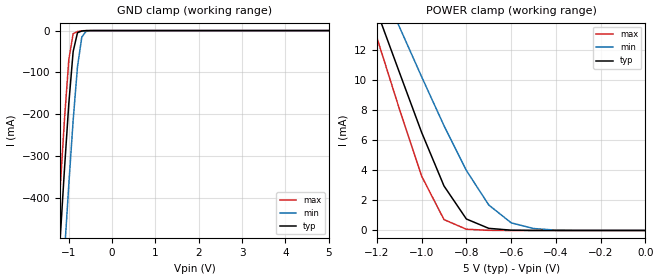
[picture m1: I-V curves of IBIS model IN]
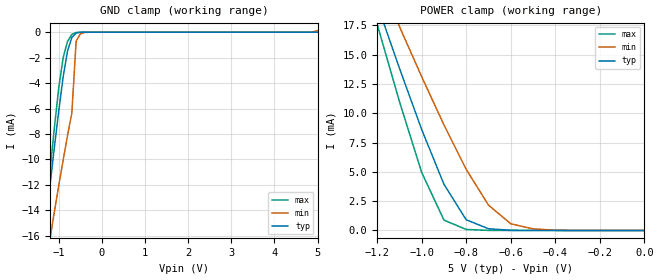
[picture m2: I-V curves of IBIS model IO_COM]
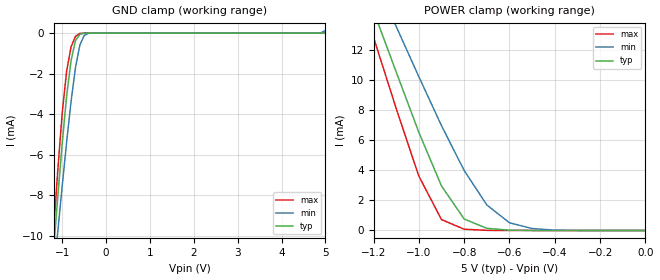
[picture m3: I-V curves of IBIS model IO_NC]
| (C) Copyright DIODES INCORPORATED
| DIODES CORPORATION
| IBIS Model of PI5A23157
| UQFN-10 (ZUA) Package
[IBIS Ver] 3.2
[Comment char] |_char
[File Name] pi5a23157_zua_50v.ibs
[File Rev] 1.0
[Source] File originated at Diodes Incorporated.
[Date] 28/11/24
[Disclaimer]
   All rights reserved
  DIODES Corporation hereby grants the user of
  this IBIS model a non-exclusive, nontransferable license to
  use this IBIS model under the following terms.
  This IBIS model is provided on an "AS IS" basis and Diodes
  makes absolutely no warranty with respect to the information
  contained herein. DIODES DISCLAIMS AND CUSTOMER WAIVES ALL
  WARRANTIES, EXPRESSED OR IMPLIED, INCLUDING WARRANTIES OF
  MERCHANTABILITY OR FITNESS FOR A PARTICULAR PURPOSE. The
  entire risk as to quality and performance is with the customer.
  Accordingly, in no event shall the company be liable for any
  damages, whether in contract or tort, including any lost
  profits or other incidental, consequential, exemplary, or
  punitive damages arising out of the use or application of the
  IBIS model provided in this package. Further, Diodes reserves
  the right to make changes without notice to any product herein
  to improve reliability, function, or design. Diodes does not
  convey any license under patent rights or any other intellectual
  property rights, including those of third parties.
  The user is granted this license only to use the IBIS model
  and is not granted rights to sell, load, rent, lease or license
  the IBIS model in whole or in part, or in modified form to anyone
  other than user. User may modify the IBIS model to suit its specific
  application but rights to derivative works and such modifications
  shall belong to Diodes.
  Diodes is not obligated to provide maintenance or support
  for the licensed IBIS model.
  Contact Diodes at ATTN: APPLICATION ENGINEERING / IBIS MODELS
  1545 Barber Lane Milpitas, CA 95035 USA.
[Component] PI5A23157
[Manufacturer] DIODES CORPORATION
[Package]
|   typ   min   max
R_pkg   50m   45m   55m
L_pkg   1.2n   1.08n   1.32n
C_pkg   0.35p   0.315p   0.385p
[Pin]   signal_name   model_name
1   IN1   IN
2   NO1   IO_NO
3   GND   GND
4   NO2   IO_NO
5   IN2   IN
6   COM2   IO_COM
7   NC2   IO_NC
8   VDD   POWER
9   NC1   IO_NC
10   COM1   IO_COM
[Series Switch Groups]
On   1 /   |NC1 to COM1
On   2 /   |NC2 to COM2
On   3 /   |NO1 to COM1
On   4 /   |NO2 to COM2
On   1 2 /
On   3 4 /
On   1 4 /
On   2 3 /
[Series Pin Mapping]   pin_2   model_name   function_table_group
9   10   SW_50   1
7   6   SW_50   2
2   10   SW_50   3
4   6   SW_50   4
[Model] SW_50
Model_type   Series_switch
Polarity   Non-Inverting
Enable  Active-High
C_comp   7.641pF   7.536pF   7.856pF
[Voltage Range]   5   4.5   5.5
[Temperature Range]   25   -40   125
[On]
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[off]
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| Models and submodels in the file (5): IN (Input), IO_COM (Terminator), IO_NC (Terminator), IO_NO (Terminator), SW_50 (Series_switch)
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[Model]   IN
Polarity   Non-Inverting
Model_type   Input
Vinl=1.50
Vinh=3.50
C_comp   1.924pF   1.914pF   1.933pF
[Voltage Range]   5   4.5   5.5
[Temperature Range]   25   -40   125
[GND Clamp Reference]   0   0   0
[POWER Clamp Reference]   5   4.5   5.5
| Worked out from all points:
|   GND clamp passes 1 mA (typ) near -0.69 V on its own axis
|   POWER clamp passes 1 mA (typ) near -0.81 V on its own axis
[GND_Clamp]
-5V       -7.41A     -7.551A    -7.332A
-1.3V     -672mA     -874.9mA   -551.1mA
-1.2V     -498.6mA   -701.3mA   -377.7mA
-1.1V     -330.7mA   -531.4mA   -212.2mA
-1V       -174.4mA   -367.4mA   -69.35mA
-900mV    -50.06mA   -214.6mA   -7.417mA
-800mV    -5.194mA   -86.41mA   -2.283mA
-700mV    -1.045mA   -15.38mA   -516.4uA
-600mV    -172uA     -1.514mA   -42.54uA
-400mV    -922.3nA   -18.02uA   -37.97nA
5V        182.5pA    1.646nA    180pA
[Power_Clamp]
|   X   TYP   MIN   MAX
-5V       91.73mA    74.17mA    111.3mA
-1.3V     18.55mA    20.11mA    17.36mA
-1.2V     14.63mA    16.91mA    12.87mA
-1.1V     10.57mA    13.6mA     8.134mA
-1V       6.542mA    10.25mA    3.625mA
-900mV    2.968mA    6.985mA    725.8uA
-800mV    765.1uA    4mA        83.69uA
-700mV    142.5uA    1.7mA      7.895uA
-600mV    19.39uA    512.9uA    574.3nA
-500mV    1.925uA    130.5uA    24.51nA
-400mV    133.8nA    21.07uA    2.542nA
0V        766.7pA    5.617nA    835.8pA
[Model]   IO_COM
Model_type   Terminator
C_comp   7.641pF   7.536pF   7.895pF
[Voltage Range]   5   4.5   5.5
[Temperature Range]   25   -40   125
[GND Clamp Reference]   0   0   0
[POWER Clamp Reference]   5   4.5   5.5
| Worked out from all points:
|   GND clamp passes 1 mA (typ) near -0.75 V on its own axis
|   POWER clamp passes 1 mA (typ) near -0.80 V on its own axis
[GND_Clamp]
-5V       -17.15A    -16.22A    -18.02A
-1.4V     -17.75mA   -25.26mA   -17.59mA
-1.3V     -14.79mA   -18.93mA   -14.14mA
-1.2V     -11.84mA   -16.13mA   -10.71mA
-1V       -6.081mA   -11.99mA   -4.28mA
-900mV    -3.48mA    -10.02mA   -1.986mA
-800mV    -1.485mA   -8.123mA   -723.2uA
-700mV    -410.4uA   -6.351mA   -175.2uA
-600mV    -64.86uA   -700.6uA   -15.81uA
-500mV    -5.833uA   -124uA     -626.8nA
-400mV    -349.8nA   -12.18uA   -15.54nA
5V        1.038nA    135uA      538.3pA
[Power_Clamp]
-5V       252.8mA    195.7mA    315.7mA
-1.2V     19.28mA    21.75mA    17.59mA
-1.1V     13.84mA    17.39mA    11mA
-1V       8.603mA    13.11mA    4.949mA
-900mV    3.939mA    8.997mA    885.1uA
-800mV    910.6uA    5.206mA    85.97uA
-700mV    147.4uA    2.162mA    8.007uA
-600mV    19.72uA    572.3uA    581nA
-500mV    1.95uA     135uA      24.84nA
-400mV    135.6nA    21.49uA    2.568nA
0V        1.039nA    6.027nA    1.119nA
[Model]   IO_NC
Model_type   Terminator
C_comp   2.888pF   2.868pF   2.934pF
[Voltage Range]   5   4.5   5.5
[Temperature Range]   25   -40   125
[GND Clamp Reference]   0   0   0
[POWER Clamp Reference]   5   4.5   5.5
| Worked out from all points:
|   GND clamp passes 1 mA (typ) near -0.76 V on its own axis
|   POWER clamp passes 1 mA (typ) near -0.81 V on its own axis
[GND_Clamp]
-5V       -8.922A    -8.398A    -9.402A
-1.2V     -10.73mA   -12.06mA   -9.815mA
-1.1V     -8.002mA   -9.748mA   -6.689mA
-1V       -5.402mA   -7.504mA   -3.897mA
-900mV    -3.084mA   -5.355mA   -1.856mA
-800mV    -1.348mA   -3.375mA   -678.2uA
-700mV    -375.7uA   -1.713mA   -162uA
-600mV    -59.31uA   -592.2uA   -14.43uA
-500mV    -5.325uA   -108.5uA   -563.8nA
-400mV    -316.6nA   -10.9uA    -13.88nA
4.8V      505.7pA    2.336uA    421.1pA
5V        764.9pA    130.5uA    480.2pA
[Power_Clamp]
-5V       91.54mA    67.74mA    111.4mA
-1.3V     18.55mA    20.11mA    17.36mA
-1.2V     14.63mA    16.91mA    12.87mA
-1.1V     10.57mA    13.6mA     8.134mA
-1V       6.542mA    10.25mA    3.625mA
-900mV    2.968mA    6.985mA    725.8uA
-800mV    765.1uA    4mA        83.69uA
-700mV    142.5uA    1.7mA      7.895uA
-600mV    19.39uA    512.9uA    574.3nA
-500mV    1.925uA    130.5uA    24.51nA
-400mV    133.8nA    21.07uA    2.542nA
0V        766.7pA    5.617nA    835.8pA
